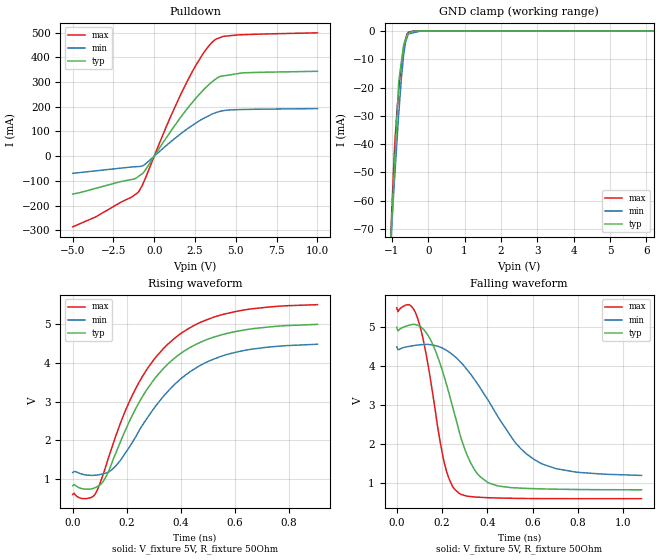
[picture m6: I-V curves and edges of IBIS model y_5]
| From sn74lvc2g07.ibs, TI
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|   y_5 Model
[Model]   y_5
Model_type   Open_drain
Polarity   Non-Inverting
Vmeas = 2.5
Vref = 5
Cref = 2pF
Rref = 1200
|   typ   min   max
|   (nom PVT)   (fast PVT)   (slow PVT)
|C_comp from frequency sweep method (F=5MHz)
C_comp   3.796e-12   3.695e-12   3.989e-12
|ON state : BUFFER OUTPUT TURNED LOW
|C_comp   3.796e-12   3.695e-12   3.989e-12
|OFF state: BUFFER IN HIGH IMPEDANCE
|C_comp   3.242e-12   3.227e-12   3.249e-12
|C_comp from LC tank measurement(L=1nH)
|Resonant Frequency(Hz)   2.780e+09   2.830e+09   2.600e+09
|C_comp   3.281e-12   3.166e-12   3.751e-12
|ON state : BUFFER OUTPUT TURNED LOW
|Resonant Frequency(Hz)   2.780e+09   2.830e+09   2.600e+09
|C_comp   3.281e-12   3.166e-12   3.751e-12
|OFF state: BUFFER IN HIGH IMPEDANCE
|Resonant Frequency(Hz)   2.820e+09   2.820e+09   2.820e+09
|C_comp   3.188e-12   3.188e-12   3.188e-12
| Where nom  PVT is Nominal Process, 5V, 27C
|   Fast PVT is Strong Process,  5.5V, -40C
|   Slow PVT is Weak Process,   4.5V, 125C
[Voltage Range]   5   4.5   5.5
|Ambient Temperature   25   85   -40
|Junction Temperature
[Temperature Range]   27   125   -40
[Pullup Reference]   5   4.5   5.5
[Pulldown Reference]   0   0   0
[Power Clamp Reference]   5   4.5   5.5
[GND Clamp Reference]   0   0   0
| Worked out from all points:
|   slope of the pulldown table from 0 to 0.75 V, typ, clamps not added: 9.97 ohm
|   GND clamp passes 1 mA (typ) near -0.56 V on its own axis
|   falling waveform, V_fixture 5V, R_fixture 50Ohm: 20-80 % time 129ps typ, 232ps min, 84.9ps max; typ from 5 V to 0.828 V
|   rising waveform, V_fixture 5V, R_fixture 50Ohm: 20-80 % time 225ps typ, 234ps min, 224ps max; typ from 0.828 V to 4.99 V
[Pulldown]
|   Voltage   I(typ)   I(min)   I(max)
-5V       -153.8mA   -69.64mA   -286.2mA
-3.586V   -130.4mA   -59.55mA   -245.9mA
-1.14V    -90.41mA   -42.87mA   -154.1mA
-995.5mV  -83.46mA   -42.3mA    -147.2mA
-670mV    -67.81mA   -38.08mA   -108.5mA
968mV     96.38mA    55.69mA    154.9mA
2.095V    198.1mA    113.4mA    312.6mA
3.08V     272.4mA    154.7mA    423.2mA
3.762V    311.8mA    176mA      472.7mA
4.218V    324.4mA    183.8mA    484.6mA
5.43V     337.1mA    188.7mA    491.4mA
10V       343.3mA    192.3mA    499mA
[GND Clamp]
|   Voltage   I(typ)   I(min)   I(max)
-5V       -1.507A    -1.223A    -1.778A
-1.058V   -80.55mA   -81.72mA   -82.53mA
-1.001V   -66.26mA   -69.21mA   -63.35mA
-907.5mV  -42.62mA   -48.96mA   -37.56mA
-858mV    -30.1mA    -38.94mA   -28.13mA
-810mV    -17.96mA   -29.36mA   -21.36mA
-738mV    -11.06mA   -16.95mA   -11.99mA
-670.5mV  -4.754mA   -8mA       -5.37mA
-616.5mV  -2.67mA    -3.587mA   -2.704mA
-544.5mV  -849uA     -1.012mA   -394.4uA
-202.5mV  -16.77uA   -369.7nA   -1.794uA
10V       0A         0A         0A
[POWER Clamp]
|   Voltage   I(typ)   I(min)   I(max)
-5V       0A         0A         0A
0V        0A         0A         0A
10V       0A         0A         0A
[Ramp]
R_load = 1200
|   typ   min   max
dV/dt_r   2.97207/5.31593e-09   2.65912/5.32529e-09   3.27942/5.29171e-09
dV/dt_f   2.97612/1.14858e-10   2.66294/1.98371e-10   3.28367/7.68564e-11
[Falling Waveform]
V_fixture = 5V
V_fixture_min = 4.5V
V_fixture_max = 5.5V
R_fixture = 50Ohm
|   Time   V(typ)   V(min)   V(max)
0s        5V         4.5V       5.5V
55ps      5.055V     4.512V     5.58V
90ps      5.06V      4.544V     5.266V
130ps     4.862V     4.563V     4.292V
210ps     3.72V      4.442V     1.512V
275ps     2.338V     4.147V     739.1mV
370ps     1.155V     3.427V     634.4mV
520ps     879.3mV    2.064V     608.4mV
605ps     857.8mV    1.613V     603.2mV
1.08ns    827.8mV    1.198V     600.4mV
[Rising Waveform]
V_fixture = 5V
V_fixture_min = 4.5V
V_fixture_max = 5.5V
R_fixture = 50Ohm
|   Time   V(typ)   V(min)   V(max)
0s        828.4mV    1.167V     600.8mV
75ps      755.6mV    1.095V     546.7mV
110ps     912.3mV    1.128V     1.063V
160ps     1.679V     1.342V     2.125V
235ps     2.843V     2.114V     3.362V
305ps     3.607V     2.867V     4.124V
385ps     4.167V     3.495V     4.679V
470ps     4.522V     3.926V     5.036V
575ps     4.767V     4.224V     5.28V
905ps     4.992V     4.479V     5.501V
